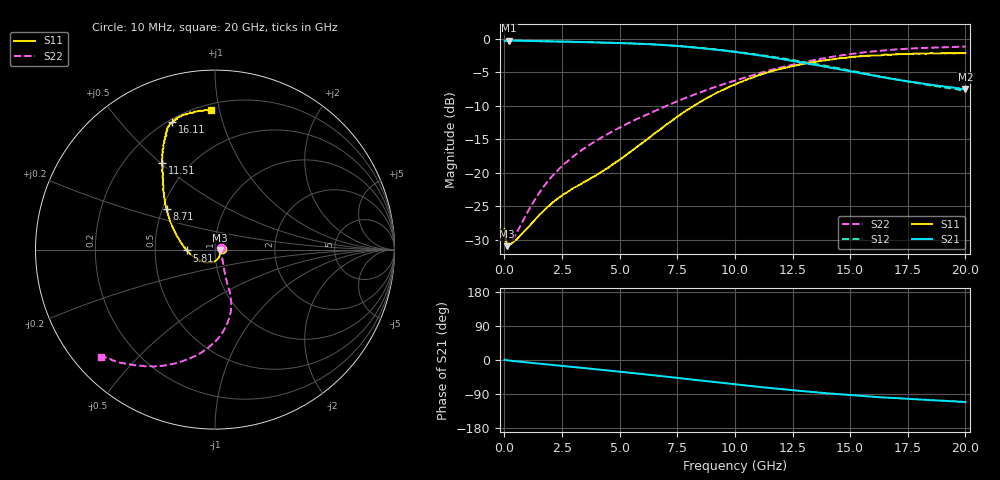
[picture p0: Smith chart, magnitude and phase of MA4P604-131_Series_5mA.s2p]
! AWR Design Environment (9226) Thu Aug 19 15:08:55 2021
! Document = '5mA'
! nPorts: 2, nXvals: 201
# GHz S DB R 50
!Freq DBS11 AngS11 DBS21 AngS21 DBS12 AngS12 DBS22 AngS22
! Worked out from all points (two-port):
!   201 points, 10 MHz to 20 GHz, reference 50 ohm
!   highest |S21| = -0.30 dB at 210 MHz (marker M1); lowest = -7.6 dB at 20 GHz (marker M2)
!   |S21| within 3 dB of the highest: start of sweep to 12.45 GHz
!   lowest |S11| = -31.0 dB at 110 MHz (marker M3), VSWR 1.06, Z = 52.9 - j0.276 ohm
!   |S11| at or under -10 dB: start of sweep to 8.237 GHz
!   |S22| runs from -31.0 to -1.2 dB; largest |S21 - S12| = 0.026
!   S11 on the Smith chart (normalised r, x): 10 MHz: 1.08, +0.01; 5.81 GHz: 0.73, -0.01; 8.71 GHz: 0.53, +0.27; 11.51 GHz: 0.36, +0.50; 16.11 GHz: 0.22, +0.70; 20 GHz: 0.24, +0.94
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0.01  -28.38 7.0  -0.38 0.9  -0.35 0.9  -29.04 17.4
0.11  -30.98 -5.3  -0.31 -0.7  -0.29 -0.7  -30.97 -6.7
0.21  -30.82 -9.5  -0.30 -1.4  -0.29 -1.4  -30.60 -11.7
0.51  -30.02 -23.0  -0.32 -3.4  -0.30 -3.3  -29.11 -27.3
1.31  -27.10 -56.2  -0.38 -8.4  -0.36 -8.2  -24.11 -50.4
1.81  -25.34 -73.3  -0.42 -11.4  -0.40 -11.1  -21.61 -57.7
2.51  -23.39 -94.5  -0.46 -15.5  -0.45 -15.2  -18.98 -64.2
3.41  -21.51 -119.0  -0.53 -21.0  -0.51 -20.5  -16.52 -67.8
4.71  -18.75 -153.1  -0.65 -28.9  -0.63 -28.3  -13.81 -70.1
5.81  -16.01 -178.4  -0.78 -35.9  -0.76 -35.1  -11.91 -71.1
6.71  -13.69 164.8  -0.93 -41.9  -0.91 -41.0  -10.54 -72.6
7.81  -10.92 149.2  -1.20 -49.4  -1.18 -48.2  -8.93 -75.8
8.71  -9.04 139.9  -1.49 -55.4  -1.45 -54.1  -7.77 -79.9
10.01  -6.85 129.2  -2.00 -64.3  -1.94 -62.6  -6.28 -87.0
11.51  -4.98 121.5  -2.76 -73.9  -2.65 -72.1  -4.74 -97.7
13.41  -3.51 115.2  -3.89 -84.5  -3.73 -83.4  -3.23 -111.6
15.01  -2.76 111.5  -4.90 -92.5  -4.77 -91.7  -2.33 -122.2
16.11  -2.51 108.5  -5.59 -97.5  -5.51 -96.6  -1.88 -127.7
16.71  -2.43 106.8  -5.96 -99.8  -5.92 -99.0  -1.70 -130.1
18.21  -2.25 102.2  -6.76 -104.5  -6.84 -104.4  -1.40 -134.7
19.51  -2.21 95.7  -7.33 -108.8  -7.53 -108.2  -1.26 -136.3
20  -2.16 91.8  -7.57 -110.9  -7.81 -109.7  -1.20 -136.7
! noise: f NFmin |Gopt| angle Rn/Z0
0.01  0  1  0  2e-20
2.21  0  1  0  2e-20
4.41  0  1  0  2e-20
6.61  0  1  0  2e-20
8.81  0  1  0  2e-20
11.11  0  1  0  2e-20
13.31  0  1  0  2e-20
15.51  0  1  0  2e-20
17.71  0  1  0  2e-20
20  0  1  0  2e-20
